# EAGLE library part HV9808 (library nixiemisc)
The HV9808 HV serial to parallel controller
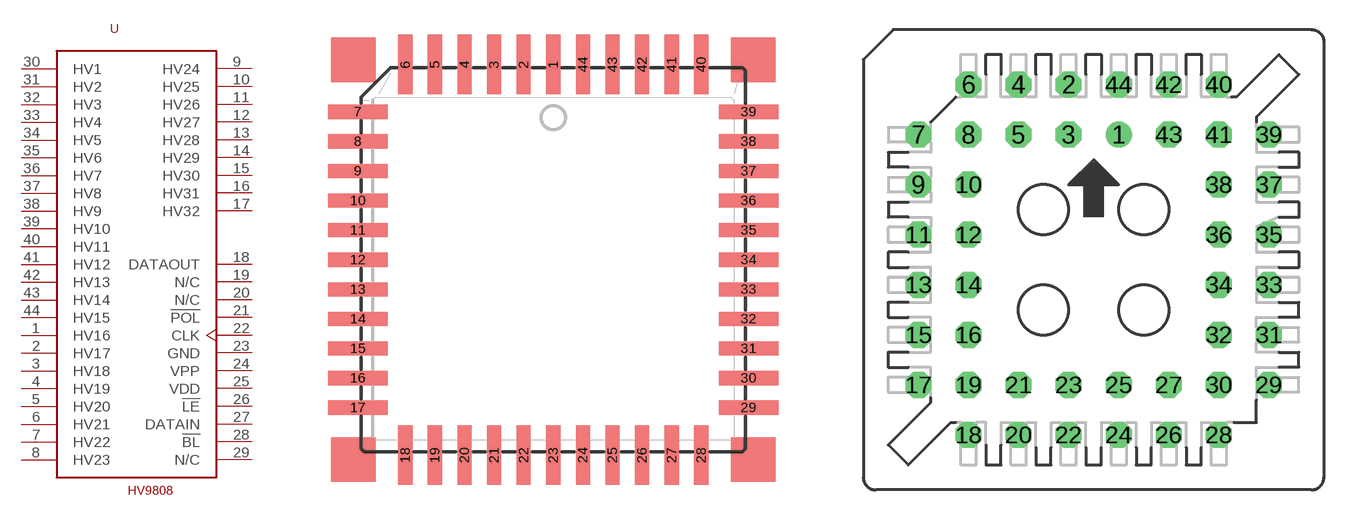
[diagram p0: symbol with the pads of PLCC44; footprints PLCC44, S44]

Designator prefix U

## HV9808PADS  [PLCC44]
1  HV16  out
2  HV17  out
3  HV18  out
4  HV19  out
5  HV20  out
6  HV21  out
7  HV22  out
8  HV23  out
9  HV24  out
10  HV25  out
11  HV26  out
12  HV27  out
13  HV28  out
14  HV29  out
15  HV30  out
16  HV31  out
17  HV32  out
18  DATAOUT  out
19  N/C  nc
20  N/C  nc
21  !POL  in
22  CLK  out
23  GND  pwr
24  VPP  pwr
25  VDD  pwr
26  !LE  in
27  DATAIN  in
28  !BL  in
29  N/C  nc
30  HV1  out
31  HV2  out
32  HV3  out
33  HV4  out
34  HV5  out
35  HV6  out
36  HV7  out
37  HV8  out
38  HV9  out
39  HV10  out
40  HV11  out
41  HV12  out
42  HV13  out
43  HV14  out
44  HV15  out

## HV9808SOCKET  [S44]
Pads as for PLCC44

## Footprint PLCC44 (pad centres in mm)
PLASTIC LEADED CHIP CARRIER square
smd 0.61 x 2.54: 1 0,8.382; 2 -1.27,8.382; 3 -2.54,8.382; 4 -3.81,8.382; 5 -5.08,8.382; 6 -6.35,8.382; 18 -6.35,-8.382; 19 -5.08,-8.382; 20 -3.81,-8.382; 21 -2.54,-8.382; 22 -1.27,-8.382; 23 0,-8.382; 24 1.27,-8.382; 25 2.54,-8.382; 26 3.81,-8.382; 27 5.08,-8.382; 28 6.35,-8.382; 40 6.35,8.382; 41 5.08,8.382; 42 3.81,8.382; 43 2.54,8.382; 44 1.27,8.382
smd 2.54 x 0.61: 7 -8.382,6.35; 8 -8.382,5.08; 9 -8.382,3.81; 10 -8.382,2.54; 11 -8.382,1.27; 12 -8.382,0; 13 -8.382,-1.27; 14 -8.382,-2.54; 15 -8.382,-3.81; 16 -8.382,-5.08; 17 -8.382,-6.35; 29 8.382,-6.35; 30 8.382,-5.08; 31 8.382,-3.81; 32 8.382,-2.54; 33 8.382,-1.27; 34 8.382,0; 35 8.382,1.27; 36 8.382,2.54; 37 8.382,3.81; 38 8.382,5.08; 39 8.382,6.35

## Footprint S44 (pad centres in mm)
PLCC SOCKET
drill 0.813: 1 1.27,6.35
drill 0.813 octagon: 2 -1.27,8.89; 3 -1.27,6.35; 4 -3.81,8.89; 5 -3.81,6.35; 6 -6.35,8.89; 7 -8.89,6.35; 8 -6.35,6.35; 9 -8.89,3.81; 10 -6.35,3.81; 11 -8.89,1.27; 12 -6.35,1.27; 13 -8.89,-1.27; 14 -6.35,-1.27; 15 -8.89,-3.81; 16 -6.35,-3.81; 17 -8.89,-6.35; 18 -6.35,-8.89; 19 -6.35,-6.35; 20 -3.81,-8.89; 21 -3.81,-6.35; 22 -1.27,-8.89; 23 -1.27,-6.35; 24 1.27,-8.89; 25 1.27,-6.35; 26 3.81,-8.89; 27 3.81,-6.35; 28 6.35,-8.89; 29 8.89,-6.35; 30 6.35,-6.35; 31 8.89,-3.81; 32 6.35,-3.81; 33 8.89,-1.27; 34 6.35,-1.27; 35 8.89,1.27; 36 6.35,1.27; 37 8.89,3.81; 38 6.35,3.81; 39 8.89,6.35; 40 6.35,8.89; 41 6.35,6.35; 42 3.81,8.89; 43 3.81,6.35; 44 1.27,8.89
